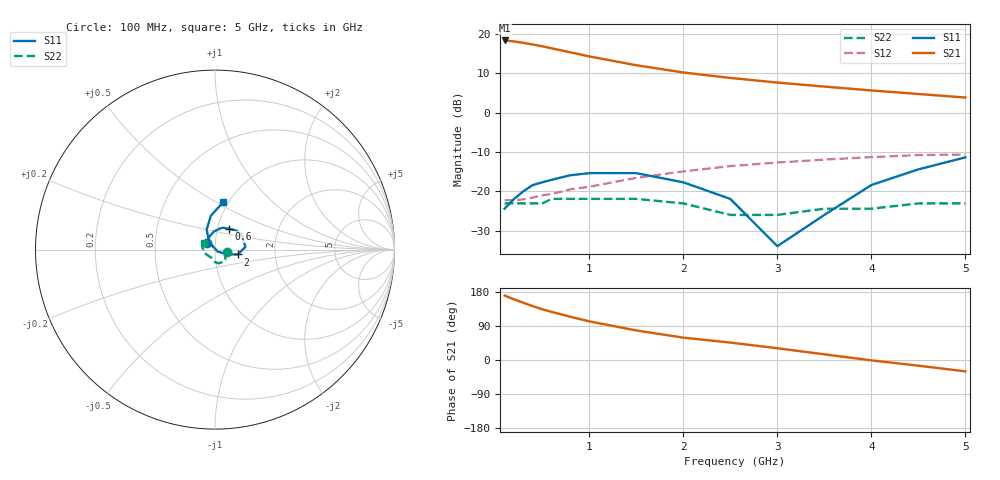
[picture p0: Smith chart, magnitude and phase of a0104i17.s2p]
!  MSA0104 S AND NOISE PARAMETERS
!  Id=17mA  LAST UPDATED 07-22-92
# ghz s ma r 50
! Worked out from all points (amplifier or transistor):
!   16 points, 100 MHz to 5 GHz, reference 50 ohm
!   highest |S21| = 18.4 dB at 100 MHz (marker M1)
!   |S21| within 3 dB of that: start of sweep to 796.2 MHz
!   unconditionally stable (mu >= 1): start of sweep to end of sweep
!   at 300 MHz: K = 1.11, MAG = 17.9 dB, |S12| = -22.0 dB
!   at 1.5 GHz: K = 1.12, MAG = 12.2 dB, |S12| = -16.6 dB
!   at 5 GHz: K = 1.23, MAG = 4.3 dB, |S12| = -10.6 dB
!   lowest NFmin = 5.20 dB at 100 MHz
!   S11 on the Smith chart (normalised r, x): 100 MHz: 0.91, +0.07; 600 MHz: 1.14, +0.27; 2 GHz: 1.29, -0.07; 5 GHz: 0.95, +0.54
0.1  0.06 141.0  8.31 170.0  0.077 5.0  0.07 -9.0
0.2  0.08 112.0  8.07 160.0  0.077 9.0  0.07 -15.0
0.3  0.1 94.0  7.75 151.0  0.079 15.0  0.07 -22.0
0.4  0.12 77.0  7.38 142.0  0.083 16.0  0.07 -32.0
0.5  0.13 70.0  7.01 134.0  0.089 19.0  0.07 -37.0
0.6  0.14 56.0  6.6 127.0  0.092 21.0  0.08 -44.0
0.8  0.16 41.0  5.87 114.0  0.106 27.0  0.08 -53.0
1  0.17 28.0  5.21 102.0  0.114 29.0  0.08 -61.0
1.5  0.17 5.0  4.02 78.0  0.148 30.0  0.08 -73.0
2  0.13 -12.0  3.25 59.0  0.179 25.0  0.07 -90.0
2.5  0.08 -20.0  2.77 46.0  0.209 25.0  0.05 -112.0
3  0.02 -37.0  2.42 31.0  0.232 18.0  0.05 -134.0
3.5  0.05 128.0  2.15 15.0  0.253 10.0  0.06 -160.0
4  0.12 113.0  1.92 -1.0  0.272 2.0  0.06 -175.0
4.5  0.19 97.0  1.73 -15.0  0.289 -7.0  0.07 173.0
5  0.27 80.0  1.56 -30.0  0.294 -15.0  0.07 150.0
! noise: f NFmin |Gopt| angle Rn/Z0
0.1  5.2  0.24  3  1.15
0.5  5.3  0.24  11  1.14
1  5.5  0.22  21  1.1
2  6  0.18  40  0.99
